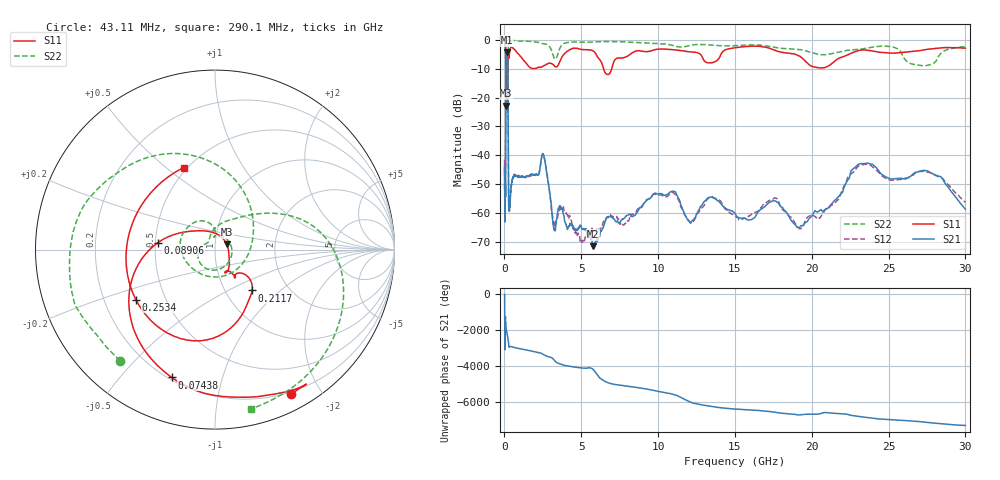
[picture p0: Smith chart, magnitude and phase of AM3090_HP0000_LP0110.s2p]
! Date/Time: Thu, Feb 28, 2019 1:53 PM
! Network Analyzer: Agilent Technologies E8364B Rev: A.07.50.67
! Sweep from 0.010 to 30.000 GHz, 1601 Points, Sweep Type: LOG
! Power Supply: 5.023 V, 0.002 A
# Hz S DB R 50
!freq MagS11 AngS11 MagS21 AngS21 MagS12 AngS12 MagS22 AngS22
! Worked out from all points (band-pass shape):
!   1601 points, 10 MHz to 30 GHz, reference 50 ohm
!   highest |S21| = -4.23 dB at 144 MHz (marker M1); lowest = -71.6 dB at 5.754 GHz (marker M2)
!   |S21| within 3 dB of the highest: 99.08 MHz to 210.3 MHz (111.2 MHz wide, 71.9 % of centre)
!   lowest |S11| = -22.9 dB at 97.46 MHz (marker M3), VSWR 1.16, Z = 56.9 + j3.36 ohm
!   |S11| at or under -10 dB: 89.16 MHz to 213.2 MHz (124 MHz wide, 82 % of centre); 6.454 GHz to 6.981 GHz (526.7 MHz wide, 7.84 % of centre)
!   |S22| runs from -25.1 to -0.2 dB; largest |S21 - S12| = 0.013
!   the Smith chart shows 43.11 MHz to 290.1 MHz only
!   S11 on the Smith chart (normalised r, x): 43.11 MHz: 0.17, -1.65; 74.38 MHz: 0.21, -0.70; 89.06 MHz: 0.51, +0.04; 211.7 MHz: 1.33, -0.67; 253.4 MHz: 0.34, -0.26; 290.1 MHz: 0.48, +0.58
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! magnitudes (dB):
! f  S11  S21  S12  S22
! 10 MHz  -0.2  -46.8  -41.5  -0.6
! 38.04 MHz  -0.5  -60.5  -60.5  -1.4
! 43.11 MHz  -0.8  -61.4  -59.1  -1.8
! 48.61 MHz  -0.9  -48.8  -47.9  -1.6
! 74.38 MHz  -2.5  -46.5  -45.7  -4.4
! 89.06 MHz  -9.8  -15.4  -15.4  -16.1
! 97.46 MHz  -22.9  -7.8  -7.8  -14.0
! 144 MHz  -15.2  -4.2  -4.2  -20.9
! 144.7 MHz  -15.2  -4.2  -4.2  -20.8
! 211.7 MHz  -10.2  -7.5  -7.5  -17.0
! 253.4 MHz  -5.7  -47.4  -47.3  -1.9
! 290.1 MHz  -6.2  -57.2  -57.6  -0.8
! 550.5 MHz  -2.8  -47.6  -47.8  -0.3
! 2.084 GHz  -9.8  -46.5  -46.8  -0.7
! 2.533 GHz  -9.0  -39.6  -39.9  -1.3
! 3.22 GHz  -8.8  -65.9  -63.3  -6.1
! 5.754 GHz  -3.7  -71.6  -65.8  -0.7
! 7.926 GHz  -5.9  -61.2  -63.7  -0.7
! 10.7 GHz  -3.3  -53.2  -53.8  -1.6
! 19.31 GHz  -6.0  -64.4  -65.4  -3.4
! 23.48 GHz  -3.5  -42.9  -43.1  -2.9
! 30 GHz  -2.8  -58.7  -56.4  -2.3
